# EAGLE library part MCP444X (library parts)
Digitalpotentiometer mit I²C, 129, TSSOP-20
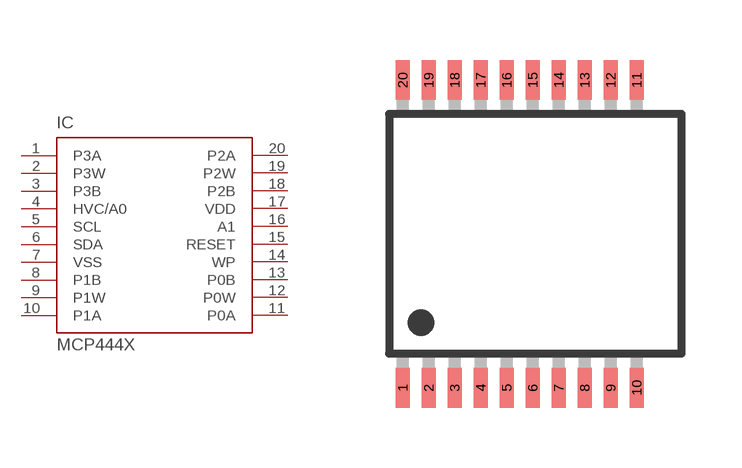
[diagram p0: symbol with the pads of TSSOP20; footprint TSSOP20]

Designator prefix IC

## MCP444X  [TSSOP20]
1  P3A  in
2  P3W  pwr
3  P3B
4  HVC/A0  pwr
5  SCL
6  SDA
7  VSS  in
8  P1B
9  P1W
10  P1A
11  P0A
12  P0W
13  P0B
14  WP
15  RESET
16  A1
17  VDD
18  P2B
19  P2W
20  P2A

## Footprint TSSOP20 (pad centres in mm)
TSSOP 20
smd 0.35 x 1: 1 -5.85,-3.85; 2 -5.2,-3.85; 3 -4.55,-3.85; 4 -3.9,-3.85; 5 -3.25,-3.85; 6 -2.6,-3.85; 7 -1.95,-3.85; 8 -1.3,-3.85; 9 -0.65,-3.85; 10 0,-3.85; 11 0,3.85; 12 -0.65,3.85; 13 -1.3,3.85; 14 -1.95,3.85; 15 -2.6,3.85; 16 -3.25,3.85; 17 -3.9,3.85; 18 -4.55,3.85; 19 -5.2,3.85; 20 -5.85,3.85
